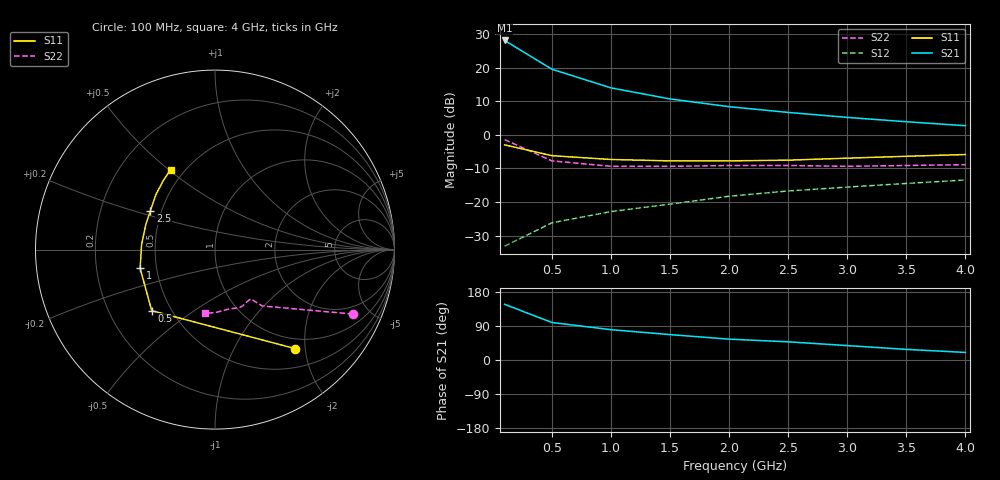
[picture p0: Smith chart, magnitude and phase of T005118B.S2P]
!AT-00511
!S-PARAMETERS at Vce=8V  Ic=15mA.  LAST UPDATED 07-21-92
!OBSOLETED Feb 1994 - nearest replacement: AT-41511
# ghz s ma r 50
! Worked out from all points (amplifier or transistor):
!   9 points, 100 MHz to 4 GHz, reference 50 ohm
!   highest |S21| = 28.1 dB at 100 MHz (marker M1)
!   |S21| within 3 dB of that: start of sweep to 240.2 MHz
!   unconditionally stable (mu >= 1): 944.8 MHz to end of sweep
!   at 500 MHz: K = 0.73, MSG = 22.9 dB, |S12| = -26.2 dB
!   at 2 GHz: K = 1.16, MAG = 10.9 dB, |S12| = -18.3 dB
!   at 4 GHz: K = 1.12, MAG = 6.0 dB, |S12| = -13.4 dB
!   S11 on the Smith chart (normalised r, x): 100 MHz: 0.81, -1.81; 500 MHz: 0.39, -0.35; 1 GHz: 0.40, -0.10; 2.5 GHz: 0.43, +0.23; 4 GHz: 0.42, +0.51
0.1  0.71 -51.0  25.48 147.0  0.022 70.0  0.85 -25.0
0.5  0.49 -136.0  9.51 99.0  0.049 50.0  0.41 -50.0
1  0.43 -166.0  5.01 80.0  0.072 52.0  0.34 -54.0
1.5  0.41 176.0  3.43 67.0  0.093 53.0  0.34 -58.0
2  0.41 160.0  2.63 55.0  0.122 54.0  0.35 -64.0
2.5  0.42 149.0  2.16 48.0  0.146 53.0  0.35 -68.0
3  0.45 137.0  1.82 38.0  0.167 52.0  0.34 -76.0
3.5  0.48 127.0  1.57 28.0  0.189 49.0  0.35 -89.0
4  0.51 119.0  1.37 20.0  0.213 45.0  0.36 -99.0
